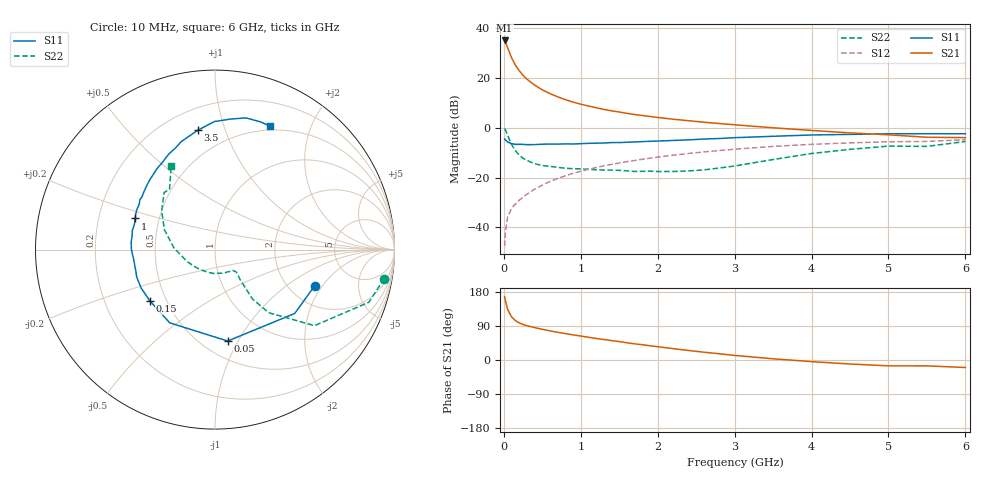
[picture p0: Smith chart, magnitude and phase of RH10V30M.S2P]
! SIEMENS Small Signal Semiconductors
! BFR106
! Si NPN RF Bipolar Junction Transistor in SOT23
! VCE = 10 V  IC = 30 mA
! Common Emitter S-Parameters:  August  1996
# GHz  S  MA  R  50
!  f  S11  S21  S12  S22
! GHz  MAG  ANG  MAG  ANG  MAG  ANG  MAG  ANG
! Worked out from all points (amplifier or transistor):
!   36 points, 10 MHz to 6 GHz, reference 50 ohm
!   highest |S21| = 35.0 dB at 10 MHz (marker M1)
!   |S21| within 3 dB of that: start of sweep to 50.05 MHz
!   unconditionally stable (mu >= 1): 328.2 MHz to 2.176 GHz
!   at 250 MHz: K = 0.93, MSG = 24.4 dB, |S12| = -27.9 dB
!   at 1.4 GHz: K = 1.06, MAG = 9.2 dB, |S12| = -14.7 dB
!   at 6 GHz: K = 0.98, MSG = 0.4 dB, |S12| = -4.8 dB
!   S11 on the Smith chart (normalised r, x): 10 MHz: 2.74, -1.69; 50 MHz: 0.65, -0.91; 150 MHz: 0.41, -0.29; 1 GHz: 0.36, +0.16; 3.5 GHz: 0.33, +0.81; 6 GHz: 0.45, +1.44
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0.01  0.5912 -19.9  56.09 167.2  0.0042 83.5  0.9569 -9.7
0.02  0.5691 -38.7  52.73 157.0  0.0082 73.0  0.906 -18.9
0.05  0.5142 -82.1  39.73 133.2  0.0163 61.7  0.6977 -37.4
0.1  0.4797 -121.7  25.37 113.9  0.024 55.9  0.4615 -49.6
0.15  0.4619 -141.9  17.93 103.8  0.0295 58.0  0.3448 -52.8
0.2  0.4638 -152.4  13.87 98.1  0.035 60.5  0.2841 -51.8
0.25  0.4623 -160.5  11.19 93.6  0.0403 62.9  0.2427 -50.8
0.3  0.4562 -165.9  9.397 90.6  0.0464 65.1  0.2205 -50.2
0.4  0.4574 -174.1  7.14 85.6  0.0583 67.7  0.1895 -47.8
0.5  0.4659 179.8  5.734 81.0  0.0704 68.4  0.1739 -46.6
0.6  0.4691 175.0  4.814 76.9  0.0835 68.7  0.1672 -46.9
0.8  0.4729 166.9  3.651 69.7  0.1085 68.1  0.1535 -49.5
1  0.4774 158.7  2.958 63.2  0.1337 67.0  0.1493 -53.6
1.1  0.4847 155.7  2.718 60.0  0.1461 66.2  0.1462 -57.2
1.3  0.4921 149.1  2.323 54.0  0.1714 64.0  0.1412 -63.0
1.6  0.5097 141.2  1.934 45.5  0.2082 60.6  0.1361 -75.7
2.2  0.5544 125.8  1.476 30.1  0.2804 53.1  0.1322 -107.3
2.8  0.6059 111.6  1.211 16.5  0.3476 44.7  0.1549 -147.2
3.5  0.6715 98.3  0.994 3.2  0.421 34.7  0.2295 177.6
4.5  0.7328 83.1  0.785 -10.6  0.495 19.7  0.3675 143.9
5.5  0.7554 70.3  0.642 -15.5  0.5299 9.0  0.421 127.0
6  0.7533 66.2  0.631 -19.8  0.5739 1.6  0.528 117.5
